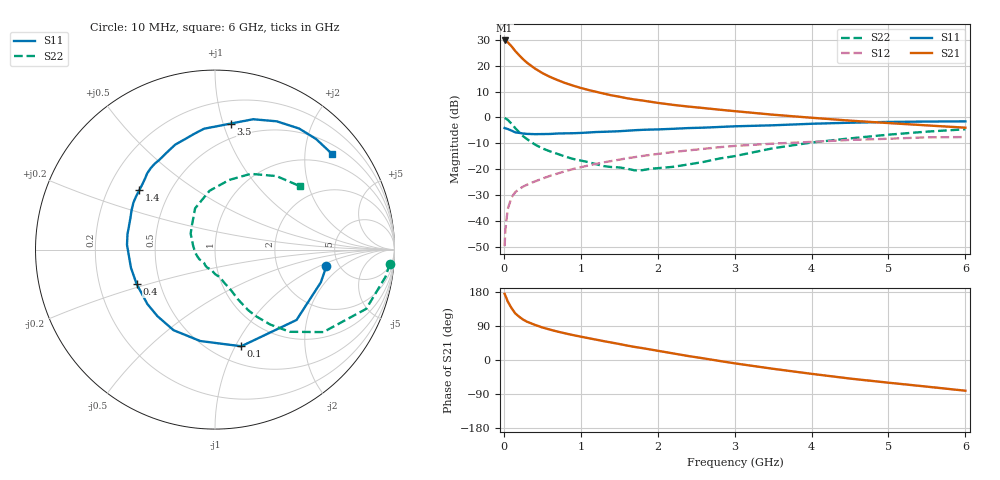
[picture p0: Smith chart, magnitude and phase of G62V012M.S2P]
! SIEMENS Small Signal Semiconductors
! BFG193
! Si NPN RF Bipolar Junction Transistor in SOT223
! VCE = 2 V  IC = 12 mA
! Common Emitter S-Parameters:  August  1996
# GHz  S  MA  R  50
!  f  S11  S21  S12  S22
! GHz  MAG  ANG  MAG  ANG  MAG  ANG  MAG  ANG
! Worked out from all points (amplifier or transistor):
!   36 points, 10 MHz to 6 GHz, reference 50 ohm
!   highest |S21| = 29.7 dB at 10 MHz (marker M1)
!   |S21| within 3 dB of that: start of sweep to 120 MHz
!   unconditionally stable (mu >= 1): 811.9 MHz to 2.686 GHz
!   at 250 MHz: K = 0.60, MSG = 24.6 dB, |S12| = -26.7 dB
!   at 1.4 GHz: K = 1.07, MAG = 11.1 dB, |S12| = -16.8 dB
!   at 6 GHz: K = 0.91, MSG = 1.8 dB, |S12| = -7.5 dB
!   S11 on the Smith chart (normalised r, x): 10 MHz: 3.96, -1.23; 100 MHz: 0.68, -1.06; 400 MHz: 0.37, -0.18; 1.4 GHz: 0.33, +0.31; 3.5 GHz: 0.38, +1.06; 6 GHz: 0.72, +2.64
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0.01  0.6274 -8.6  30.6 174.5  0.0033 91.4  0.9771 -4.6
0.02  0.6172 -17.2  30.17 170.1  0.0068 86.2  0.9625 -9.0
0.05  0.6001 -40.8  28.26 154.7  0.017 72.6  0.9048 -21.4
0.1  0.5581 -74.8  23.62 136.9  0.0288 61.8  0.7585 -37.3
0.15  0.5159 -99.2  19.02 122.7  0.0365 54.7  0.6192 -47.7
0.2  0.505 -117.2  15.83 114.1  0.0418 52.4  0.5189 -53.6
0.25  0.4903 -130.9  13.32 106.6  0.0464 50.3  0.4372 -58.3
0.3  0.4836 -141.2  11.43 101.2  0.0505 50.6  0.3844 -61.3
0.4  0.477 -156.2  8.88 93.0  0.0582 51.0  0.3036 -65.3
0.5  0.4791 -167.8  7.202 85.9  0.0662 51.2  0.2537 -67.8
0.6  0.4814 -176.3  6.075 80.2  0.0749 51.9  0.2223 -70.3
0.7  0.491 176.9  5.252 74.9  0.0832 51.9  0.1982 -73.5
0.9  0.4971 164.4  4.118 65.7  0.1014 50.8  0.1589 -79.1
1.1  0.5136 154.9  3.391 57.6  0.1188 49.5  0.1376 -89.3
1.4  0.5362 141.8  2.676 46.0  0.1447 45.0  0.1108 -107.0
1.7  0.5684 131.7  2.224 34.5  0.172 40.5  0.0957 -130.0
2.2  0.6053 116.0  1.752 17.4  0.2158 30.4  0.1119 -172.1
2.8  0.6564 99.9  1.416 -2.4  0.2672 17.7  0.1615 147.0
3.5  0.7076 82.9  1.132 -23.2  0.3132 1.2  0.2553 115.7
4.5  0.7932 64.3  0.87 -49.0  0.3696 -18.5  0.3955 78.6
5.5  0.8347 47.6  0.704 -70.3  0.4151 -41.9  0.534 50.1
6  0.8425 39.1  0.636 -81.1  0.4193 -55.4  0.592 36.5
